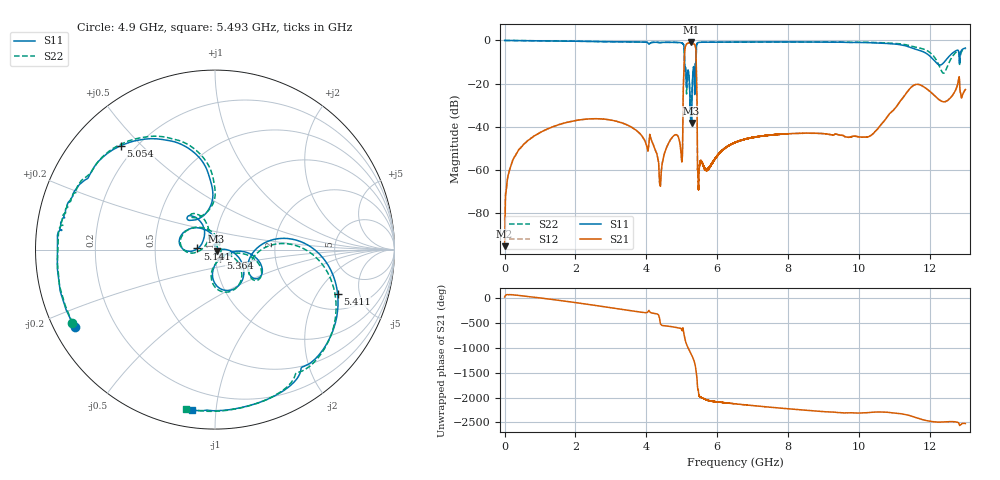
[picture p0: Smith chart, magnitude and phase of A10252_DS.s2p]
!Akoustis s2p Touchstone File
!Script Version: 1.0
!Creation Data: 4/14/2021 at 11:44 AM
!DEEMBEDDING STATE: ON
!DEMBEDDING OFFSET: 0.3 dB static
! Freq Mag(S11) Angle(S11)Mag(S21) Angle(S21)Mag(S12) Angle(S12)Mag(S22) Angle(S22)
# GHz S MA R 50
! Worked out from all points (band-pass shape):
!   11000 points, 1 MHz to 13 GHz, reference 50 ohm
!   highest |S21| = -0.94 dB at 5.25 GHz (marker M1); lowest = -95.4 dB at 1 MHz (marker M2)
!   |S21| within 3 dB of the highest: 5.087 GHz to 5.395 GHz (308.3 MHz wide, 5.88 % of centre)
!   lowest |S11| = -38.3 dB at 5.276 GHz (marker M3), VSWR 1.02, Z = 50.8 - j0.897 ohm
!   |S11| at or under -10 dB: 5.079 GHz to 5.4 GHz (321.2 MHz wide, 6.13 % of centre); 12.16 GHz to 12.4 GHz (247.9 MHz wide, 2.02 % of centre); 12.82982 GHz to 12.83853 GHz (8.714 MHz wide, 0.0679 % of centre)
!   |S22| runs from -32.8 to 0.0 dB; largest |S21 - S12| = 0.0019
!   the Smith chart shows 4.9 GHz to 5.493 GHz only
!   S11 on the Smith chart (normalised r, x): 4.9 GHz: 0.06, -0.26; 5.054 GHz: 0.15, +0.44; 5.141 GHz: 0.82, +0.01; 5.364 GHz: 1.05, -0.10; 5.411 GHz: 2.92, -3.06; 5.493 GHz: 0.09, -0.86
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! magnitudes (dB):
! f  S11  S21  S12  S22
! 1 MHz  0.0  -95.4  -83.6  0.0
! 26.12 MHz  0.0  -72.2  -70.7  0.0
! 126.6 MHz  0.0  -61.0  -60.4  0.0
! 553.7 MHz  -0.1  -47.9  -47.9  -0.1
! 2.689 GHz  -0.5  -36.3  -36.3  -0.5
! 4.9 GHz  -1.0  -44.6  -44.6  -1.0
! 5.009 GHz  -1.2  -54.7  -54.8  -1.2
! 5.054 GHz  -2.1  -16.7  -16.7  -2.2
! 5.087 GHz  -14.2  -3.9  -3.9  -13.9
! 5.141 GHz  -20.2  -1.6  -1.6  -21.7
! 5.193 GHz  -15.0  -1.1  -1.1  -15.2
! 5.25 GHz  -37.5  -0.9  -0.9  -29.2
! 5.276 GHz  -38.3  -1.0  -1.0  -27.8
! 5.321 GHz  -13.4  -1.4  -1.4  -13.2
! 5.364 GHz  -24.9  -1.9  -1.8  -24.4
! 5.411 GHz  -2.8  -13.8  -13.7  -2.8
! 5.454 GHz  -1.0  -61.4  -61.5  -1.0
! 5.493 GHz  -0.9  -59.4  -59.3  -0.9
! 6.836 GHz  -0.7  -45.5  -45.6  -0.8
! 10.14 GHz  -1.0  -44.8  -44.9  -0.8
! 11.54 GHz  -3.8  -20.8  -20.8  -2.9
! 13 GHz  -3.5  -22.7  -22.7  -3.7
